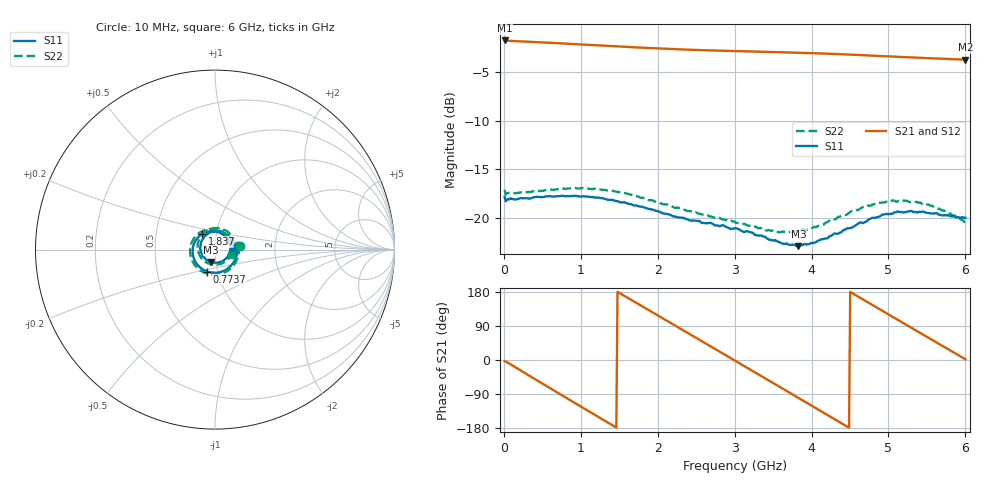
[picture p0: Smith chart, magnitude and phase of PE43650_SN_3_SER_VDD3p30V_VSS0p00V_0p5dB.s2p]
!Keysight Technologies,N5245B,MY57181451,A.13.50.07
!Date: Tuesday, May 07, 2019 07:59:45
!Correction: S11(Full 2 Port(1,2))
!S21(Full 2 Port(1,2))
!S12(Full 2 Port(1,2))
!S22(Full 2 Port(1,2))
!S2P File: Measurements: S11, S21, S12, S22:
# Hz S  dB  R 50
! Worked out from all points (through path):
!   401 points, 10 MHz to 6 GHz, reference 50 ohm
!   highest |S21| = -1.75 dB at 10 MHz (marker M1); lowest = -3.7 dB at 6 GHz (marker M2)
!   group delay of S21, straight-line fit = 331 ps
!   lowest |S11| = -22.9 dB at 3.829 GHz (marker M3), VSWR 1.15, Z = 47.5 - j6.52 ohm
!   |S11| at or under -10 dB: start of sweep to end of sweep
!   |S22| runs from -21.5 to -16.9 dB; largest |S21 - S12| = 0.0056
!   S11 on the Smith chart (normalised r, x): 10 MHz: 1.29, +0.06; 773.7 MHz: 0.89, -0.22; 1.837 GHz: 0.85, +0.15; 6 GHz: 1.22, -0.01
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1e7  -17.83 9.8  -1.75 -3.3  -1.80 -3.2  -17.13 9.3
2.1965e8  -17.96 -32.5  -1.85 -27.7  -1.90 -27.7  -17.40 -32.6
4.44275e8  -17.82 -64.7  -1.93 -55.2  -1.99 -55.2  -17.22 -65.4
7.73725e8  -17.72 -109.7  -2.06 -95.3  -2.11 -95.3  -16.99 -110.2
1.013325e9  -17.80 -140.4  -2.17 -124.3  -2.21 -124.3  -16.93 -141.1
1.432625e9  -18.22 171.1  -2.34 -174.7  -2.40 -174.7  -17.25 170.0
1.83695e9  -18.96 129.7  -2.51 137.0  -2.57 137.0  -18.04 127.2
2.01665e9  -19.35 112.8  -2.58 115.6  -2.63 115.7  -18.42 109.5
2.2263e9  -19.86 93.4  -2.65 90.7  -2.70 90.8  -18.96 89.1
2.450925e9  -20.27 71.9  -2.72 64.1  -2.77 64.1  -19.29 66.9
2.73545e9  -20.72 44.3  -2.79 30.3  -2.84 30.4  -19.97 37.4
3.005e9  -21.07 13.2  -2.84 -1.7  -2.90 -1.6  -20.42 6.4
3.45425e9  -22.27 -46.8  -2.93 -55.2  -2.98 -55.1  -21.28 -56.0
3.828625e9  -22.91 -107.2  -3.02 -99.8  -3.06 -99.8  -21.40 -115.0
4.008325e9  -22.58 -138.1  -3.06 -121.3  -3.10 -121.3  -21.03 -144.7
4.2629e9  -21.81 -179.8  -3.13 -151.8  -3.18 -151.7  -20.34 175.6
4.5025e9  -21.05 144.7  -3.21 179.6  -3.26 179.7  -19.41 140.8
4.7421e9  -20.14 112.1  -3.30 151.0  -3.35 151.2  -18.74 109.6
5.01165e9  -19.60 80.5  -3.39 119.0  -3.44 119.2  -18.24 76.8
5.445925e9  -19.34 36.8  -3.54 67.5  -3.59 67.6  -18.64 30.0
5.745425e9  -19.76 13.4  -3.65 32.0  -3.69 32.1  -19.33 2.4
6e9  -19.99 -3.3  -3.72 1.9  -3.77 2.0  -20.46 -17.4
